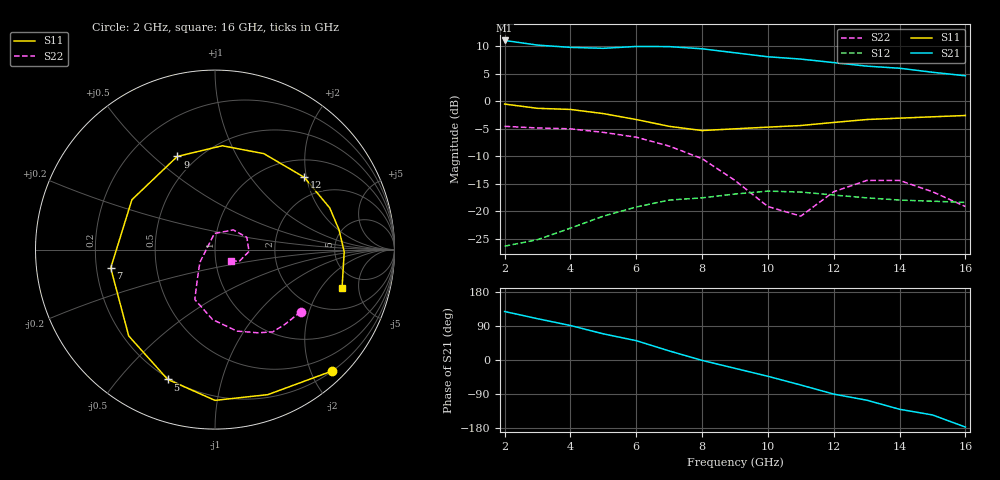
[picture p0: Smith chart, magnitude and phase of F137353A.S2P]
!ATF-13735
!S-PARAMETERS at Vds=2.5V  Id=20mA.  LAST UPDATED 07-22-92
# ghz s ma r 50
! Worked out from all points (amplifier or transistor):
!   15 points, 2 GHz to 16 GHz, reference 50 ohm
!   highest |S21| = 11.0 dB at 2 GHz (marker M1)
!   |S21| within 3 dB of that: start of sweep to 10.08 GHz
!   unconditionally stable (mu >= 1): 9.946 GHz to end of sweep
!   at 4 GHz: K = 0.60, MSG = 16.4 dB, |S12| = -23.1 dB
!   at 9 GHz: K = 0.98, MSG = 12.8 dB, |S12| = -16.9 dB
!   at 16 GHz: K = 1.22, MAG = 8.7 dB, |S12| = -18.4 dB
!   lowest NFmin = 1.00 dB at 2 GHz
!   S11 on the Smith chart (normalised r, x): 2 GHz: 0.20, -2.34; 5 GHz: 0.19, -0.68; 7 GHz: 0.26, -0.08; 9 GHz: 0.40, +0.60; 12 GHz: 1.42, +1.94; 16 GHz: 3.42, -3.27
2  0.94 -46.0  3.56 128.0  0.048 55.0  0.59 -36.0
3  0.86 -70.0  3.23 109.0  0.055 40.0  0.57 -47.0
4  0.84 -90.0  3.08 91.0  0.07 31.0  0.56 -55.0
5  0.77 -110.0  3.02 69.0  0.09 18.0  0.52 -63.0
6  0.68 -135.0  3.14 51.0  0.109 7.0  0.47 -75.0
7  0.59 -170.0  3.13 24.0  0.126 -12.0  0.39 -92.0
8  0.54 149.0  2.99 -1.0  0.132 -27.0  0.3 -112.0
9  0.56 112.0  2.75 -22.0  0.143 -43.0  0.19 -121.0
10  0.58 86.0  2.53 -43.0  0.152 -58.0  0.11 -140.0
11  0.6 63.0  2.41 -66.0  0.149 -73.0  0.09 92.0
12  0.64 39.0  2.24 -90.0  0.14 -81.0  0.15 47.0
13  0.68 20.0  2.08 -106.0  0.132 -90.0  0.19 21.0
14  0.7 9.0  1.99 -130.0  0.126 -97.0  0.19 -3.0
15  0.72 -1.0  1.83 -145.0  0.123 -111.0  0.15 -26.0
16  0.74 -17.0  1.7 -177.0  0.12 -129.0  0.11 -34.0
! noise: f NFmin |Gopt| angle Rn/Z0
2  1  0.84  51  0.38
4  1.1  0.71  102  0.1
6  1.3  0.55  147  0.07
8  1.5  0.46  -144  0.19
12  1.8  0.5  -40  0.88
14  2.1  0.52  -4  1.17
